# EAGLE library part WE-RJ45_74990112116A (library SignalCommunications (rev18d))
Order Code 74990112116A Design THT xBase-T 10/100 Base-T Ports 1x1 Application Standard Tab Position UP LED (Left-Right) Green-Yellow EMI Fingers Yes Details see: http://katalog.we-online.de/en/pbs/WE-LAN_RJ45/74990112116A? Updated by Yingchun Shan 2016-08-29 2016(C) Würth Elektronik
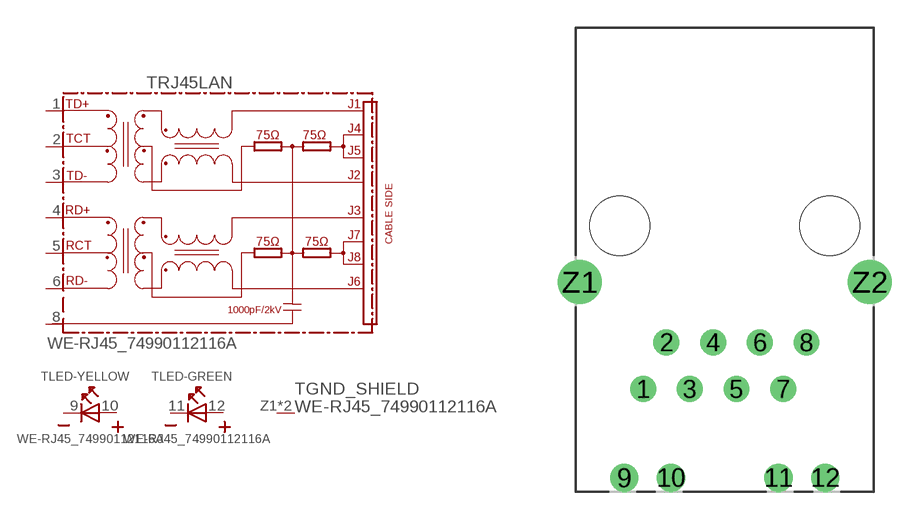
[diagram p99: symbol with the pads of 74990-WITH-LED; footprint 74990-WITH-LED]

Designator prefix T; gates RJ45LAN=74990X-THT-10/100-T LED-GREEN=LED2PIN LED-YELLOW=LED2PIN GND_SHIELD=GND_PIN

## WE-RJ45_74990112116A (COMPANY-URL: http://www.we-online.de; CREATED-BY: Christin Zierenner; CREATED-DATE: AUG 2012; DATASHEET-URL: http://katalog.we-online.de/kataloge/eisos/media/pdf/74990112116A.pdf; MANUFACTURER: Würth Elektronik eiSos GmbH)  [74990-WITH-LED]
1  RJ45LAN:TD+
2  RJ45LAN:TCT
3  RJ45LAN:TD-
4  RJ45LAN:RD+
5  RJ45LAN:RCT
6  RJ45LAN:RD-
8  RJ45LAN:8
9  LED-YELLOW:K  pas
10  LED-YELLOW:A  pas
11  LED-GREEN:K  pas
12  LED-GREEN:A  pas
Z1  GND_SHIELD:1  pwr
Z2  GND_SHIELD:1  pwr

## Footprint 74990-WITH-LED (pad centres in mm)
MAX HEIGHT=13.50mm PORTS----1X1 LED -YES
drill 0.9: 1 -4.445,-8.89; 2 -3.175,-6.35; 3 -1.905,-8.89; 4 -0.635,-6.35; 5 0.635,-8.89; 6 1.905,-6.35; 7 3.175,-8.89; 8 4.445,-6.35
drill 1.02: 9 -5.465,-13.72; 10 -2.925,-13.72; 11 2.925,-13.72; 12 5.465,-13.72
drill 1.6: Z1 -7.9,-3.05; Z2 7.9,-3.05
hole 3.25 at -5.715,0
hole 3.25 at 5.715,0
